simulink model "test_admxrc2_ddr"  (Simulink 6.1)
settings: Solver=ode45  StartTime=0.0  StopTime=400  RelTol=1e-3
undefined symbols (not defined in the file or in its folder): Bit, Location, Lower, netlist, Width
libraries: xbsIndex_r3 x84, adlibrary2 x4

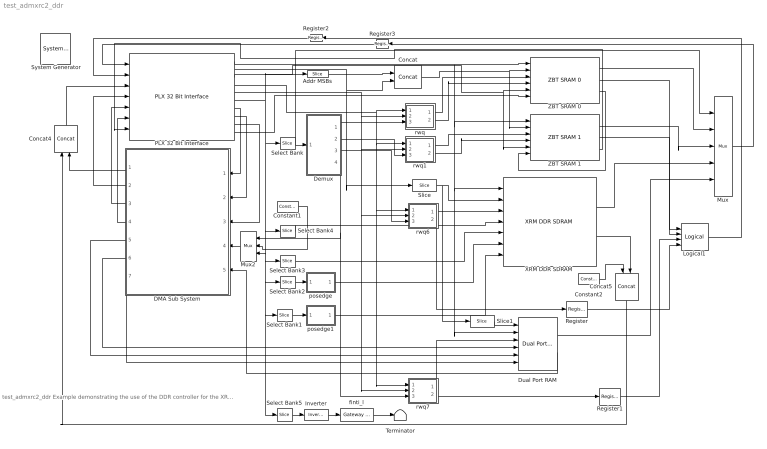
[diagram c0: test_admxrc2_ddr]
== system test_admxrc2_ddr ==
  note: test_admxrc2_ddr Example demonstrating the use of the DDR controller for the XRM-DDR-IO module
  " System Generator" : xbsIndex_r3/ System Generator  Tag=genX  xilinxfamily=Virtex2  part=xc2v3000  speed=-4  package=ff1152  synthesis_tool=XST  directory=./netlist  testbench=off  simulink_period=1  sysclk_period=10  incr_netlist=off  trim_vbits=Everywhere in SubSystem  dbl_ovrd=According to Block Masks  core_generation=According to Block Masks  run_coregen=off  deprecated_control=off  eval_field=0
  Addr MSBs : xbsIndex_r3/Slice  mode=Lower Bit Location + Width  nbits=4  bit1=0  base1=MSB of Input  bit0=4  base0=LSB of Input  boolean_output=off  explicit_period=on  period=1  dbl_ovrd=off
  Concat : xbsIndex_r3/Concat  num_inputs=2  explicit_period=on  period=1  dbl_ovrd=off
  Concat4 : xbsIndex_r3/Concat  Orientation=up  num_inputs=2  explicit_period=on  period=1  dbl_ovrd=off
  Concat5 : xbsIndex_r3/Concat  Orientation=down  num_inputs=2  explicit_period=on  period=1  dbl_ovrd=off
  Constant1 : xbsIndex_r3/Constant  const=0  equ=P=C  arith_type=Unsigned  n_bits=32  bin_pt=0  opselect=C  inp2=PCIN>>17  opr=+  inp1=P  carry=CIN  iostate=0  explicit_period=off  period=1  dbl_ovrd=off
  Constant2 : xbsIndex_r3/Constant  const=0  equ=P=C  arith_type=Unsigned  n_bits=3  bin_pt=0  opselect=C  inp2=PCIN>>17  opr=+  inp1=P  carry=CIN  iostate=0  explicit_period=off  period=1  dbl_ovrd=off
  DMA Sub System : Subsystem  Orientation=left
  Demux : Subsystem
  Dual Port RAM : xbsIndex_r3/Dual Port RAM  depth=1024  initVector=sin(pi*(0:15)/16)  write_mode_A=Read After Write  write_mode_B=Read After Write  latency=1  mem_collision=off  init_zero=on  explicit_period=on  period=1  dbl_ovrd=off  rst_a=off  init_a=0  rst_b=off  init_b=0  show_param=off  distributed_mem=off  use_rpm=off  gen_core=off
  Inverter : xbsIndex_r3/Inverter  latency=0  explicit_period=off  period=1  en=off  dbl_ovrd=off  show_param=off
  Logical1 : xbsIndex_r3/Logical  logical_function=OR  inputs=4  precision=Full  arith_type=Unsigned  n_bits=8  bin_pt=2  align_bp=off  latency=0  explicit_period=off  period=1  en=off  dbl_ovrd=off  show_param=off
  Mux : xbsIndex_r3/Mux  inputs=4  precision=Full  arith_type="Signed  (2's comp)"  n_bits=8  bin_pt=2  quantization=Truncate  overflow=Wrap  latency=0  explicit_period=off  period=1  en=off  dbl_ovrd=off  show_param=off  mux_type=off  use_rpm=off  gen_core=off
  Mux2 : xbsIndex_r3/Mux  Orientation=left  inputs=2  precision=Full  arith_type="Signed  (2's comp)"  n_bits=8  bin_pt=2  quantization=Truncate  overflow=Wrap  latency=0  explicit_period=off  period=1  en=off  dbl_ovrd=off  show_param=off  mux_type=off  use_rpm=off  gen_core=off
  PLX 32 Bit Interface : adlibrary2/ADM-XRC-II/PLX 32 Bit Interface  program='load test_admxpl_ddr_program.txt'  clock_ratio=1.5
  Register : xbsIndex_r3/Register  init=0  reg_only_valid=off  explicit_period=off  period=1  rst=off  en=off  out_en=off  dbl_ovrd=off  show_param=off
  Register1 : xbsIndex_r3/Register  init=0  reg_only_valid=off  explicit_period=off  period=1  rst=off  en=off  out_en=off  dbl_ovrd=off  show_param=off
  Register2 : xbsIndex_r3/Register  Orientation=left  init=0  reg_only_valid=off  explicit_period=on  period=1  rst=off  en=off  out_en=off  dbl_ovrd=off  show_param=off
  Register3 : xbsIndex_r3/Register  Orientation=left  init=0  reg_only_valid=off  explicit_period=on  period=1  rst=off  en=off  out_en=off  dbl_ovrd=off  show_param=off
  Select Bank : xbsIndex_r3/Slice  mode=Lower Bit Location + Width  nbits=2  bit1=0  base1=MSB of Input  bit0=0  base0=LSB of Input  boolean_output=off  explicit_period=on  period=1  dbl_ovrd=off
  Select Bank1 : xbsIndex_r3/Slice  mode=Lower Bit Location + Width  nbits=1  bit1=0  base1=MSB of Input  bit0=3  base0=LSB of Input  boolean_output=on  explicit_period=on  period=1  dbl_ovrd=off
  Select Bank2 : xbsIndex_r3/Slice  mode=Lower Bit Location + Width  nbits=1  bit1=0  base1=MSB of Input  bit0=2  base0=LSB of Input  boolean_output=on  explicit_period=on  period=1  dbl_ovrd=off
  Select Bank3 : xbsIndex_r3/Slice  mode=Lower Bit Location + Width  nbits=4  bit1=0  base1=MSB of Input  bit0=8  base0=LSB of Input  boolean_output=off  explicit_period=on  period=1  dbl_ovrd=off
  Select Bank4 : xbsIndex_r3/Slice  mode=Lower Bit Location + Width  nbits=14  bit1=0  base1=MSB of Input  bit0=16  base0=LSB of Input  boolean_output=off  explicit_period=on  period=1  dbl_ovrd=off
  Select Bank5 : xbsIndex_r3/Slice  mode=Lower Bit Location + Width  nbits=1  bit1=0  base1=MSB of Input  bit0=15  base0=LSB of Input  boolean_output=on  explicit_period=on  period=1  dbl_ovrd=off
  Slice : xbsIndex_r3/Slice  mode=Lower Bit Location + Width  nbits=11  bit1=0  base1=MSB of Input  bit0=0  base0=LSB of Input  boolean_output=off  explicit_period=on  period=1  dbl_ovrd=off
  Slice1 : xbsIndex_r3/Slice  mode=Lower Bit Location + Width  nbits=10  bit1=0  base1=MSB of Input  bit0=0  base0=LSB of Input  boolean_output=off  explicit_period=on  period=1  dbl_ovrd=off
  Terminator : Terminator
  "XRM DDR SDRAM " : adlibrary2/ADM-XRC-II/XRM DDR SDRAM   memsize=1
  ZBT SRAM 0 : adlibrary2/ADM-XRC-II/ZBT SRAM 0
  ZBT SRAM 1 : adlibrary2/ADM-XRC-II/ZBT SRAM 1
  finti_l : xbsIndex_r3/Gateway Out  output_type=Double  nbits=8  bin_pt=6  arith_type=Boolean  quantization=Truncate  overflow=Wrap  hdl_port=on  timing_constraint=None  locs_specified=on  LOCs={'AM2'}  needs_fixed_name=off  show_param=off
  posedge : Subsystem
  posedge1 : Subsystem
  rwq : Subsystem
  rwq1 : Subsystem
  rwq6 : Subsystem
  rwq7 : Subsystem
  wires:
  PLX 32 Bit Interface/1 -> ZBT SRAM 0/1, Dual Port RAM/2, "XRM DDR SDRAM "/1, ZBT SRAM 1/1
  Register/1 -> Logical1/4
  Register1/1 -> Logical1/3
  Mux/1 -> Register3/1
  Register2/1 -> PLX 32 Bit Interface/2
  Register3/1 -> PLX 32 Bit Interface/1
  Slice/1 -> Slice1/1, "XRM DDR SDRAM "/2
  Addr MSBs/1 -> Concat/1
  PLX 32 Bit Interface/2 -> Concat/2, Slice/1
  Select Bank/1 -> Demux/1(Select), Mux/1
  rwq6/1(wq) -> "XRM DDR SDRAM "/3
  rwq6/2(rq) -> Register/1
  rwq7/1(wq) -> Dual Port RAM/3
  rwq7/2(rq) -> Register1/1
  Demux/1(En0) -> rwq/3(e)
  Demux/2(En1) -> rwq1/3(e)
  DMA Sub System/2(Read IFIFO) -> PLX 32 Bit Interface/4
  DMA Sub System/3(Write OFIFO) -> PLX 32 Bit Interface/5
  DMA Sub System/4(OFIFO_Data) -> PLX 32 Bit Interface/6
  Dual Port RAM/2 -> DMA Sub System/5(DP_RAM_Data)
  DMA Sub System/7(DP_RAM_WE) -> Dual Port RAM/6
  DMA Sub System/6(DP_RAM_Addr) -> Dual Port RAM/4
  DMA Sub System/5(DP_RAM_WData) -> Dual Port RAM/5
  Logical1/1 -> Register2/1
  rwq/1(wq) -> ZBT SRAM 0/3
  rwq1/1(wq) -> ZBT SRAM 1/3
  rwq/2(rq) -> ZBT SRAM 0/4
  rwq1/2(rq) -> ZBT SRAM 1/4
  Demux/3(En2) -> rwq6/3(e)
  Demux/4(En3) -> rwq7/3(e), Mux2/1
  "XRM DDR SDRAM "/1 -> Mux/4
  Dual Port RAM/1 -> Mux/5
  PLX 32 Bit Interface/4 -> rwq/1(w), rwq1/1(w), rwq6/1(w), rwq7/1(w)
  PLX 32 Bit Interface/9 -> DMA Sub System/3(OFIFO_Full)
  PLX 32 Bit Interface/8 -> DMA Sub System/2(IFIFO_Empty)
  PLX 32 Bit Interface/7 -> DMA Sub System/1(IFIFO_Data)
  PLX 32 Bit Interface/6 -> Select Bank4/1, Select Bank2/1, Select Bank1/1, Select Bank5/1, Select Bank3/1, Mux2/3, Select Bank/1, Addr MSBs/1
  PLX 32 Bit Interface/5 -> rwq7/2(r), rwq6/2(r), rwq1/2(r), rwq/2(r)
  PLX 32 Bit Interface/3 -> ZBT SRAM 0/5, ZBT SRAM 1/5
  Concat4/1 -> PLX 32 Bit Interface/3
  DMA Sub System/1(Status) -> Concat4/2
  "XRM DDR SDRAM "/2 -> Concat5/2
  Concat5/1 -> Concat4/1
  posedge/1(Out1) -> "XRM DDR SDRAM "/6
  posedge1/1(Out1) -> "XRM DDR SDRAM "/7
  Select Bank2/1 -> posedge/1(In1)
  Select Bank1/1 -> posedge1/1(In1)
  Select Bank3/1 -> "XRM DDR SDRAM "/5
  Select Bank4/1 -> "XRM DDR SDRAM "/4
  Select Bank5/1 -> Inverter/1
  finti_l/1 -> Terminator/1
  Mux2/1 -> DMA Sub System/4(Control)
  Constant1/1 -> Mux2/2
  ZBT SRAM 1/2 -> Logical1/2
  ZBT SRAM 0/2 -> Logical1/1
  ZBT SRAM 1/1 -> Mux/3
  ZBT SRAM 0/1 -> Mux/2
  Concat/1 -> ZBT SRAM 0/2, ZBT SRAM 1/2
  Slice1/1 -> Dual Port RAM/1
  PLX 32 Bit Interface/10 -> ZBT SRAM 0/6
  ZBT SRAM 0/3 -> ZBT SRAM 1/6
  ZBT SRAM 1/3 -> PLX 32 Bit Interface/7
  Constant2/1 -> Concat5/1
  Inverter/1 -> finti_l/1

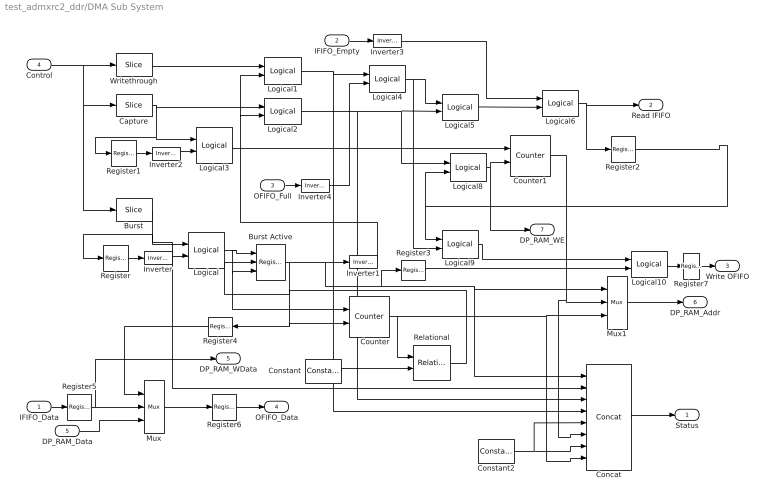
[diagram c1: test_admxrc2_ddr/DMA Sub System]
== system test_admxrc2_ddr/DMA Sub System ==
  IFIFO_Data : Inport  Port=1  LatchInput=off
  IFIFO_Empty : Inport  Port=2  LatchInput=off
  OFIFO_Full : Inport  Port=3  LatchInput=off
  Control : Inport  Port=4  LatchInput=off
  DP_RAM_Data : Inport  Port=5  LatchInput=off
  Burst : xbsIndex_r3/Slice  mode=Lower Bit Location + Width  nbits=1  bit1=0  base1=MSB of Input  bit0=6  base0=LSB of Input  boolean_output=on  explicit_period=on  period=1  dbl_ovrd=off
  Burst Active : xbsIndex_r3/Register  init=0  reg_only_valid=off  explicit_period=on  period=1  rst=on  en=on  out_en=off  dbl_ovrd=off  show_param=off
  Capture : xbsIndex_r3/Slice  mode=Lower Bit Location + Width  nbits=1  bit1=0  base1=MSB of Input  bit0=5  base0=LSB of Input  boolean_output=on  explicit_period=on  period=1  dbl_ovrd=off
  Concat : xbsIndex_r3/Concat  num_inputs=8  explicit_period=on  period=1  dbl_ovrd=off
  Constant : xbsIndex_r3/Constant  const=511  equ=P=C  arith_type=Unsigned  n_bits=10  bin_pt=0  opselect=C  inp2=PCIN>>17  opr=+  inp1=P  carry=CIN  iostate=0  explicit_period=off  period=1  dbl_ovrd=off
  Constant2 : xbsIndex_r3/Constant  const=0  equ=P=C  arith_type=Unsigned  n_bits=2  bin_pt=0  opselect=C  inp2=PCIN>>17  opr=+  inp1=P  carry=CIN  iostate=0  explicit_period=off  period=1  dbl_ovrd=off
  Counter : xbsIndex_r3/Counter  cnt_type=Count Limited  n_bits=10  bin_pt=0  arith_type=Unsigned  start_count=0  cnt_to=Inf  cnt_by_val=1  operation=Up  explicit_period=on  period=1  load_pin=off  rst=on  en=on  dbl_ovrd=off  show_param=off  use_rpm=on  gen_core=off
  Counter1 : xbsIndex_r3/Counter  cnt_type=Count Limited  n_bits=10  bin_pt=0  arith_type=Unsigned  start_count=0  cnt_to=Inf  cnt_by_val=1  operation=Up  explicit_period=on  period=1  load_pin=off  rst=on  en=on  dbl_ovrd=off  show_param=off  use_rpm=on  gen_core=off
  Inverter{,1..2,4} (4 alike) : xbsIndex_r3/Inverter  latency=0  explicit_period=off  period=1  en=off  dbl_ovrd=off  show_param=off
  Inverter3 : xbsIndex_r3/Inverter  latency=0  explicit_period=on  period=1  en=off  dbl_ovrd=off  show_param=off
  Logical : xbsIndex_r3/Logical  logical_function=AND  inputs=2  precision=Full  arith_type=Unsigned  n_bits=8  bin_pt=2  align_bp=on  latency=0  explicit_period=on  period=1  en=off  dbl_ovrd=off  show_param=off
  Logical{1..2,4,8..9} (5 alike) : xbsIndex_r3/Logical  logical_function=AND  inputs=2  precision=Full  arith_type=Unsigned  n_bits=8  bin_pt=2  align_bp=on  latency=0  explicit_period=off  period=1  en=off  dbl_ovrd=off  show_param=off
  Logical10 : xbsIndex_r3/Logical  logical_function=OR  inputs=2  precision=Full  arith_type=Unsigned  n_bits=8  bin_pt=2  align_bp=on  latency=0  explicit_period=on  period=1  en=off  dbl_ovrd=off  show_param=off
  Logical3 : xbsIndex_r3/Logical  logical_function=AND  inputs=2  precision=Full  arith_type=Unsigned  n_bits=8  bin_pt=2  align_bp=on  latency=0  explicit_period=on  period=1  en=off  dbl_ovrd=off  show_param=off
  Logical5 : xbsIndex_r3/Logical  logical_function=OR  inputs=2  precision=Full  arith_type=Unsigned  n_bits=8  bin_pt=2  align_bp=on  latency=0  explicit_period=off  period=1  en=off  dbl_ovrd=off  show_param=off
  Logical6 : xbsIndex_r3/Logical  logical_function=AND  inputs=2  precision=Full  arith_type=Unsigned  n_bits=8  bin_pt=2  align_bp=on  latency=0  explicit_period=on  period=1  en=off  dbl_ovrd=off  show_param=off
  Mux : xbsIndex_r3/Mux  inputs=2  precision=Full  arith_type="Signed  (2's comp)"  n_bits=8  bin_pt=2  quantization=Truncate  overflow=Wrap  latency=0  explicit_period=on  period=1  en=off  dbl_ovrd=off  show_param=off  mux_type=off  use_rpm=off  gen_core=off
  Mux1 : xbsIndex_r3/Mux  inputs=2  precision=Full  arith_type="Signed  (2's comp)"  n_bits=8  bin_pt=2  quantization=Truncate  overflow=Wrap  latency=0  explicit_period=off  period=1  en=off  dbl_ovrd=off  show_param=off  mux_type=off  use_rpm=off  gen_core=off
  Register{,1..3,5..7} (7 alike) : xbsIndex_r3/Register  init=0  reg_only_valid=off  explicit_period=on  period=1  rst=off  en=off  out_en=off  dbl_ovrd=off  show_param=off
  Register4 : xbsIndex_r3/Register  Orientation=left  init=0  reg_only_valid=off  explicit_period=on  period=1  rst=off  en=off  out_en=off  dbl_ovrd=off  show_param=off
  Relational : xbsIndex_r3/Relational  mode=a=b  latency=0  explicit_period=off  period=1  en=off  dbl_ovrd=off  show_param=off
  Writethrough : xbsIndex_r3/Slice  mode=Lower Bit Location + Width  nbits=1  bit1=0  base1=MSB of Input  bit0=4  base0=LSB of Input  boolean_output=on  explicit_period=on  period=1  dbl_ovrd=off
  Status : Outport
  Read IFIFO : Outport  Port=2
  Write OFIFO : Outport  Port=3
  OFIFO_Data : Outport  Port=4
  DP_RAM_WData : Outport  Port=5
  DP_RAM_Addr : Outport  Port=6
  DP_RAM_WE : Outport  Port=7
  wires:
  Mux/1 -> Register6/1
  IFIFO_Data/1 -> Register5/1
  DP_RAM_Data/1 -> Mux/3
  Control/1 -> Writethrough/1, Burst/1, Capture/1
  Burst/1 -> Register/1, Logical/1, Concat/2
  Register/1 -> Inverter/1
  Inverter/1 -> Logical/2
  Logical/1 -> Burst Active/1, Burst Active/3, Counter/1
  Burst Active/1 -> Inverter1/1, Register3/1, Mux1/1, Concat/1, Counter/2, Register4/1
  Inverter1/1 -> Logical1/2, Logical2/2
  Capture/1 -> Logical2/1, Logical3/1, Register1/1
  Writethrough/1 -> Logical1/1
  Register1/1 -> Inverter2/1
  Inverter2/1 -> Logical3/2
  Logical3/1 -> Counter1/1
  IFIFO_Empty/1 -> Inverter3/1
  OFIFO_Full/1 -> Inverter4/1
  Logical1/1 -> Logical4/1, Concat/4
  Inverter4/1 -> Logical4/2
  Logical2/1 -> Logical5/2, Logical8/1, Concat/3
  Logical4/1 -> Logical5/1, Logical9/2
  Inverter3/1 -> Logical6/1
  Logical5/1 -> Logical6/2
  Logical6/1 -> Read IFIFO/1, Register2/1
  Register2/1 -> Logical8/2, Logical9/1
  Logical8/1 -> Counter1/2, DP_RAM_WE/1
  Mux1/1 -> DP_RAM_Addr/1
  Counter1/1 -> Mux1/2, Concat/6
  Counter/1 -> Relational/1, Mux1/3, Concat/8
  Logical9/1 -> Logical10/1
  Register3/1 -> Logical10/2
  Constant/1 -> Relational/2
  Relational/1 -> Burst Active/2
  Constant2/1 -> Concat/5, Concat/7
  Concat/1 -> Status/1
  Logical10/1 -> Register7/1
  Register4/1 -> Mux/1
  Register5/1 -> Mux/2, DP_RAM_WData/1
  Register6/1 -> OFIFO_Data/1
  Register7/1 -> Write OFIFO/1

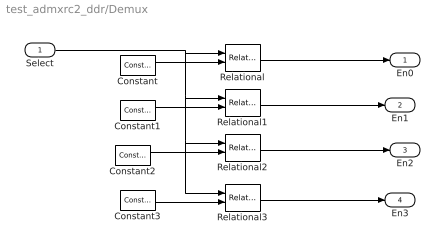
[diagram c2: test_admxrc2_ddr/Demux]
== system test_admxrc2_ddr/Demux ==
  Select : Inport  Port=1  LatchInput=off
  Constant : xbsIndex_r3/Constant  const=0  equ=P=C  arith_type=Unsigned  n_bits=2  bin_pt=0  opselect=C  inp2=PCIN>>17  opr=+  inp1=P  carry=CIN  iostate=0  explicit_period=off  period=1  dbl_ovrd=off
  Constant1 : xbsIndex_r3/Constant  const=1  equ=P=C  arith_type=Unsigned  n_bits=2  bin_pt=0  opselect=C  inp2=PCIN>>17  opr=+  inp1=P  carry=CIN  iostate=0  explicit_period=off  period=1  dbl_ovrd=off
  Constant2 : xbsIndex_r3/Constant  const=2  equ=P=C  arith_type=Unsigned  n_bits=2  bin_pt=0  opselect=C  inp2=PCIN>>17  opr=+  inp1=P  carry=CIN  iostate=0  explicit_period=off  period=1  dbl_ovrd=off
  Constant3 : xbsIndex_r3/Constant  const=3  equ=P=C  arith_type=Unsigned  n_bits=2  bin_pt=0  opselect=C  inp2=PCIN>>17  opr=+  inp1=P  carry=CIN  iostate=0  explicit_period=off  period=1  dbl_ovrd=off
  Relational{,1..3} (4 alike) : xbsIndex_r3/Relational  mode=a=b  latency=0  explicit_period=off  period=1  en=off  dbl_ovrd=off  show_param=off
  En0 : Outport
  En1 : Outport  Port=2
  En2 : Outport  Port=3
  En3 : Outport  Port=4
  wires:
  Relational/1 -> En0/1
  Relational1/1 -> En1/1
  Relational2/1 -> En2/1
  Relational3/1 -> En3/1
  Select/1 -> Relational/1, Relational1/1, Relational2/1, Relational3/1
  Constant/1 -> Relational/2
  Constant1/1 -> Relational1/2
  Constant2/1 -> Relational2/2
  Constant3/1 -> Relational3/2

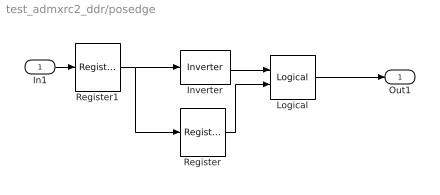
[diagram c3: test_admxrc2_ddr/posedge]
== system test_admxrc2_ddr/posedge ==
  In1 : Inport  Port=1  LatchInput=off
  Inverter : xbsIndex_r3/Inverter  latency=0  explicit_period=off  period=1  en=off  dbl_ovrd=off  show_param=off
  Logical : xbsIndex_r3/Logical  logical_function=AND  inputs=2  precision=Full  arith_type=Unsigned  n_bits=8  bin_pt=2  align_bp=on  latency=0  explicit_period=off  period=1  en=off  dbl_ovrd=off  show_param=off
  Register : xbsIndex_r3/Register  init=0  reg_only_valid=off  explicit_period=on  period=1  rst=off  en=off  out_en=off  dbl_ovrd=off  show_param=off
  Register1 : xbsIndex_r3/Register  init=0  reg_only_valid=off  explicit_period=on  period=1  rst=off  en=off  out_en=off  dbl_ovrd=off  show_param=off
  Out1 : Outport
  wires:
  Inverter/1 -> Logical/1
  Logical/1 -> Out1/1
  Register/1 -> Logical/2
  In1/1 -> Register1/1
  Register1/1 -> Inverter/1, Register/1

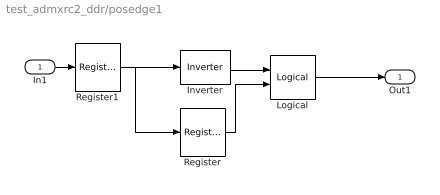
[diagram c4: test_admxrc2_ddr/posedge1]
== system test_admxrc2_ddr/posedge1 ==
  In1 : Inport  Port=1  LatchInput=off
  Inverter : xbsIndex_r3/Inverter  latency=0  explicit_period=off  period=1  en=off  dbl_ovrd=off  show_param=off
  Logical : xbsIndex_r3/Logical  logical_function=AND  inputs=2  precision=Full  arith_type=Unsigned  n_bits=8  bin_pt=2  align_bp=on  latency=0  explicit_period=off  period=1  en=off  dbl_ovrd=off  show_param=off
  Register : xbsIndex_r3/Register  init=0  reg_only_valid=off  explicit_period=on  period=1  rst=off  en=off  out_en=off  dbl_ovrd=off  show_param=off
  Register1 : xbsIndex_r3/Register  init=0  reg_only_valid=off  explicit_period=on  period=1  rst=off  en=off  out_en=off  dbl_ovrd=off  show_param=off
  Out1 : Outport
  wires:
  Inverter/1 -> Logical/1
  Logical/1 -> Out1/1
  Register/1 -> Logical/2
  In1/1 -> Register1/1
  Register1/1 -> Inverter/1, Register/1

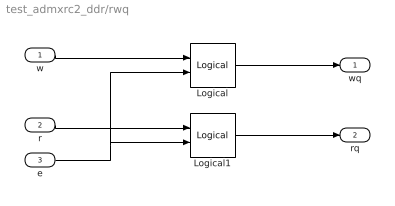
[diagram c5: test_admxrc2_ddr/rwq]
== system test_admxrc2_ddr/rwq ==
  w : Inport  Port=1  LatchInput=off
  r : Inport  Port=2  LatchInput=off
  e : Inport  Port=3  LatchInput=off
  Logical : xbsIndex_r3/Logical  logical_function=AND  inputs=2  precision=Full  arith_type=Unsigned  n_bits=8  bin_pt=2  align_bp=on  latency=0  explicit_period=off  period=1  en=off  dbl_ovrd=off  show_param=off
  Logical1 : xbsIndex_r3/Logical  logical_function=AND  inputs=2  precision=Full  arith_type=Unsigned  n_bits=8  bin_pt=2  align_bp=on  latency=0  explicit_period=off  period=1  en=off  dbl_ovrd=off  show_param=off
  wq : Outport
  rq : Outport  Port=2
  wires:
  e/1 -> Logical1/2, Logical/2
  r/1 -> Logical1/1
  w/1 -> Logical/1
  Logical/1 -> wq/1
  Logical1/1 -> rq/1

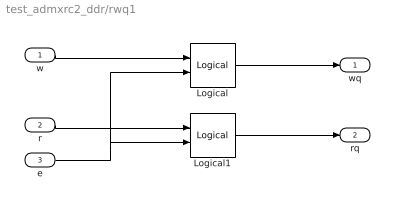
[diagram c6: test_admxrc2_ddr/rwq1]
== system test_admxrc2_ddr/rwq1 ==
  w : Inport  Port=1  LatchInput=off
  r : Inport  Port=2  LatchInput=off
  e : Inport  Port=3  LatchInput=off
  Logical : xbsIndex_r3/Logical  logical_function=AND  inputs=2  precision=Full  arith_type=Unsigned  n_bits=8  bin_pt=2  align_bp=on  latency=0  explicit_period=off  period=1  en=off  dbl_ovrd=off  show_param=off
  Logical1 : xbsIndex_r3/Logical  logical_function=AND  inputs=2  precision=Full  arith_type=Unsigned  n_bits=8  bin_pt=2  align_bp=on  latency=0  explicit_period=off  period=1  en=off  dbl_ovrd=off  show_param=off
  wq : Outport
  rq : Outport  Port=2
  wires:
  e/1 -> Logical1/2, Logical/2
  r/1 -> Logical1/1
  w/1 -> Logical/1
  Logical/1 -> wq/1
  Logical1/1 -> rq/1

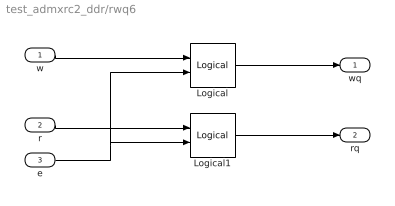
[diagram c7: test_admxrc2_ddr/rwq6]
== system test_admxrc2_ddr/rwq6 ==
  w : Inport  Port=1  LatchInput=off
  r : Inport  Port=2  LatchInput=off
  e : Inport  Port=3  LatchInput=off
  Logical : xbsIndex_r3/Logical  logical_function=AND  inputs=2  precision=Full  arith_type=Unsigned  n_bits=8  bin_pt=2  align_bp=on  latency=0  explicit_period=off  period=1  en=off  dbl_ovrd=off  show_param=off
  Logical1 : xbsIndex_r3/Logical  logical_function=AND  inputs=2  precision=Full  arith_type=Unsigned  n_bits=8  bin_pt=2  align_bp=on  latency=0  explicit_period=off  period=1  en=off  dbl_ovrd=off  show_param=off
  wq : Outport
  rq : Outport  Port=2
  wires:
  e/1 -> Logical1/2, Logical/2
  r/1 -> Logical1/1
  w/1 -> Logical/1
  Logical/1 -> wq/1
  Logical1/1 -> rq/1

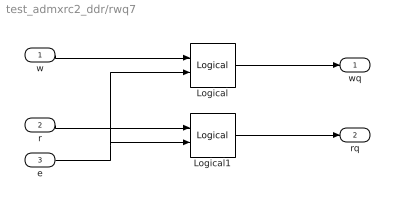
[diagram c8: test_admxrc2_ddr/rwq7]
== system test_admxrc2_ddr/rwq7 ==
  w : Inport  Port=1  LatchInput=off
  r : Inport  Port=2  LatchInput=off
  e : Inport  Port=3  LatchInput=off
  Logical : xbsIndex_r3/Logical  logical_function=AND  inputs=2  precision=Full  arith_type=Unsigned  n_bits=8  bin_pt=2  align_bp=on  latency=0  explicit_period=off  period=1  en=off  dbl_ovrd=off  show_param=off
  Logical1 : xbsIndex_r3/Logical  logical_function=AND  inputs=2  precision=Full  arith_type=Unsigned  n_bits=8  bin_pt=2  align_bp=on  latency=0  explicit_period=off  period=1  en=off  dbl_ovrd=off  show_param=off
  wq : Outport
  rq : Outport  Port=2
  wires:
  e/1 -> Logical1/2, Logical/2
  r/1 -> Logical1/1
  w/1 -> Logical/1
  Logical/1 -> wq/1
  Logical1/1 -> rq/1
